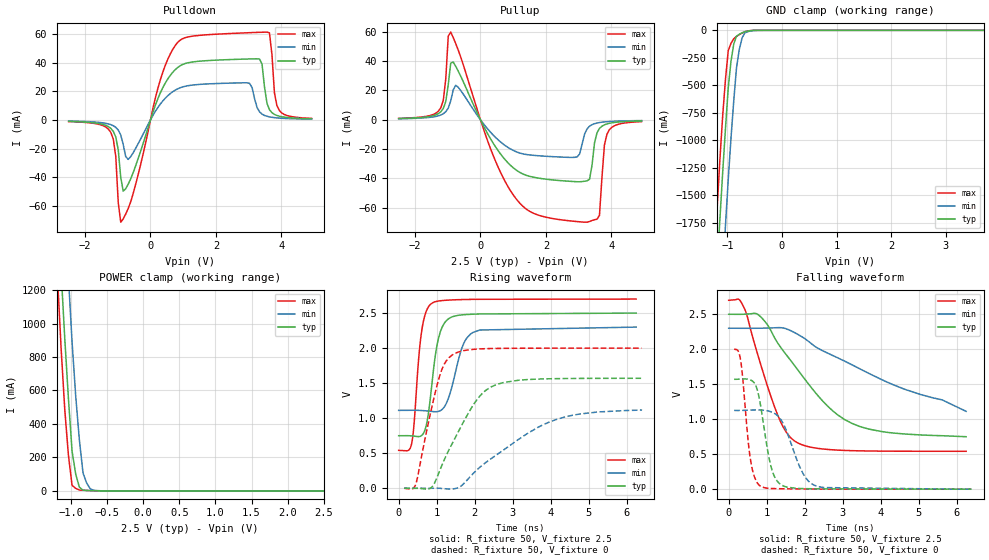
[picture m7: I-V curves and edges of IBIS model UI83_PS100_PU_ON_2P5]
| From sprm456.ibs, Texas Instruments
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|IDG09_OUI83_PS100_PU_OFF_2P75; BUFFER IN NORMAL MODE WITH PULLUP AND PU
|LLDOWN OFF
|   Model Cell UI83_PS100_PU_ON_2P5
|IDG09_OUI83_PS100_PU_ON_2P5
[Model]   UI83_PS100_PU_ON_2P5
Model_type   I/O
Polarity   Non-Inverting
Enable   Active-Low
Vinl =  0.7V
Vinh =  1.7V
Cref =  15pF
Rref =  100.00M
Vref =  0V
Vmeas =  1.25
C_comp   4.785p   4.743p   5.018p
[Model Spec]
Vinl   0.7V   0.7V   0.7V
Vinh   1.7V   1.7V   1.7V
[Temperature Range]   25   125   -40
[Voltage Range]   2.5   2.3   2.7
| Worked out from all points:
|   slope of the pulldown table from 0 to 0.375 V, typ, clamps not added: 16.7 ohm
|   slope of the pullup table from 0 to 0.375 V, typ, clamps not added: 24.3 ohm
|   GND clamp passes 1 mA (typ) near -0.53 V on its own axis
|   POWER clamp passes 1 mA (typ) near -0.67 V on its own axis
|   rising waveform, R_fixture 50, V_fixture 2.5: 20-80 % time 263ps typ, 360ps min, 200ps max; typ from 0.75 V to 2.5 V
|   rising waveform, R_fixture 50, V_fixture 0: 20-80 % time 922ps typ, 1.79ns min, 495ps max; typ from 0 V to 1.57 V
|   falling waveform, R_fixture 50, V_fixture 2.5: 20-80 % time 1.56ns typ, 2.86ns min, 775ps max; typ from 2.5 V to 0.75 V
|   falling waveform, R_fixture 50, V_fixture 0: 20-80 % time 300ps typ, 487ps min, 213ps max; typ from 1.57 V to 0 V
| Nom Voltages:
|   VDD=1.1, VDDS=2.5, VSS=0, VSSS=0
| Min Voltages:
|   VDD=1, VDDS=2.3, VSS=0, VSSS=0
| Max Voltages:
|   VDD=1.2, VDDS=2.7, VSS=0, VSSS=0
[POWER_clamp]
|   voltage   I(typ)   I(min)   I(max)
-2.5V     14.33A     15.07A     13.92A
-1.187V   1.745A     2.55A      1.279A
-1.136V   1.31A      2.108A     850.1mA
-1.086V   910.1mA    1.685A     485.5mA
-1.035V   552.6mA    1.279A     213.3mA
-984.8mV  237.5mA    889.6mA    33.3mA
-934.3mV  99.9mA     565.9mA    15.21mA
-883.8mV  22.21mA    305.1mA    5.394mA
-833.3mV  4.4mA      107.3mA    3.844mA
-732.3mV  1.653mA    12.24mA    2.077mA
-681.8mV  1.081mA    2.967mA    1.344mA
2.5V      -62.22uA   -39.52uA   -107.1uA
[Pulldown]
|   voltage   I(typ)   I(min)   I(max)
-2.5V     -1.029mA   -780.5uA   -1.158mA
-1.212V   -5.915mA   -3.318mA   -8.754mA
-1.061V   -11.95mA   -5.187mA   -25.54mA
-909.1mV  -40.09mA   -10.52mA   -71.53mA
-681.8mV  -44.99mA   -27.63mA   -62.02mA
303mV     19mA       11.15mA    28.2mA
984.8mV   38.8mA     23.1mA     56.82mA
3.03V     42.63mA    25.53mA    61mA
3.333V    42.55mA    5.654mA    61.25mA
3.636V    7.154mA    2.123mA    60.83mA
3.864V    3.092mA    1.414mA    10.01mA
4.924V    800.1uA    540.5uA    1.094mA
[Pullup]
|   voltage   I(typ)   I(min)   I(max)
-2.5V     856.4uA    691.1uA    993.5uA
-1.212V   5.469mA    3.267mA    8.206mA
-909.1mV  38.64mA    12.9mA     59.79mA
-681.8mV  33.25mA    22.23mA    47.64mA
984.8mV   -32.38mA   -20.68mA   -50.65mA
2.955V    -42.21mA   -25.24mA   -69.37mA
3.182V    -41.85mA   -9.733mA   -69.79mA
3.333V    -40.49mA   -4.356mA   -69.34mA
3.636V    -5.897mA   -1.881mA   -65.15mA
3.788V    -3.419mA   -1.448mA   -17.24mA
3.939V    -2.377mA   -1.175mA   -6.756mA
4.924V    -777.2uA   -520.7uA   -1.228mA
[GND_clamp]
|   voltage   I(typ)   I(min)   I(max)
-2.5V     -14.77A    -15.66A    -14.27A
-1.237V   -2.604A    -3.547A    -2.05A
-1.187V   -2.151A    -3.09A     -1.601A
-1.136V   -1.705A    -2.638A    -1.162A
-1.035V   -889mA     -1.772A    -443mA
-984.8mV  -521mA     -1.356A    -183.2mA
-934.3mV  -279.7mA   -978.6mA   -118.7mA
-883.8mV  -123.6mA   -639.8mA   -76.1mA
-833.3mV  -52.76mA   -339.6mA   -55.47mA
-732.3mV  -22.91mA   -70.07mA   -24.96mA
-429.3mV  -158.7uA   -473.7uA   -130.9uA
5V        0A         0A         0A
[Ramp]
| variable   typ   min   max
dV/dt_f   1.058093/1.5633404n 0.71845704/2.8620974n  1.3054833/0.77919182n
dV/dt_r 0.94951792/0.92585824n 0.68174694/1.7998433n  1.2076225/0.49653644n
R_load = 50
[Rising Waveform]
R_fixture = 50
V_fixture = 2.5
V_fixture_min = 2.3
V_fixture_max = 2.7
|   time   V(typ)   V(min)   V(max)
0s        749.7mV    1.112V     541.4mV
343.1ps   747.5mV    1.113V     640.5mV
606ps     753.9mV    1.11V      2.245V
750.2ps   960.4mV    1.103V     2.557V
910.8ps   1.665V     1.094V     2.652V
1.045ns   2.132V     1.097V     2.672V
1.197ns   2.351V     1.158V     2.681V
1.68ns    2.475V     2.025V     2.693V
1.951ns   2.484V     2.223V     2.696V
6.25ns    2.5V       2.3V       2.7V
[Rising Waveform]
R_fixture = 50
V_fixture = 0
V_fixture_min = 0
V_fixture_max = 0
|   time   V(typ)   V(min)   V(max)
143.6ps   0V         0V         0V
444.3ps   0V         0V         49.73mV
835.8ps   0V         0V         1.068V
1.045ns   203.7mV    0V         1.54V
1.205ns   412.5mV    -6.008mV   1.775V
1.453ns   684.1mV    -7.719mV   1.916V
2.086ns   1.283V     276.1mV    1.987V
2.591ns   1.483V     482.4mV    1.995V
4.15ns    1.564V     982mV      1.999V
6.394ns   1.57V      1.125V     2V
[Falling Waveform]
R_fixture = 50
V_fixture = 2.5
V_fixture_min = 2.3
V_fixture_max = 2.7
|   time   V(typ)   V(min)   V(max)
0s        2.5V       2.3V       2.7V
259.9ps   2.499V     2.3V       2.715V
411.1ps   2.501V     2.299V     2.587V
774.2ps   2.495V     2.3V       1.906V
1.226ns   2.147V     2.307V     1.15V
1.473ns   1.952V     2.299V     852.6mV
1.756ns   1.75V      2.231V     680.7mV
2.608ns   1.185V     1.944V     567.7mV
3.257ns   937.2mV    1.774V     550mV
6.25ns    749.7mV    1.112V     541.4mV
[Falling Waveform]
R_fixture = 50
V_fixture = 0
V_fixture_min = 0
V_fixture_max = 0
|   time   V(typ)   V(min)   V(max)
143.6ps   1.57V      1.125V     2V
318.1ps   1.574V     1.125V     1.83V
595.8ps   1.555V     1.131V     351.4mV
720.6ps   1.471V     1.133V     121.5mV
844.8ps   1.179V     1.132V     39.46mV
1.134ns   285.6mV    1.101V     9.611mV
1.461ns   41.36mV    909.2mV    5.33mV
1.909ns   9.314mV    274mV      3.042mV
2.274ns   5.385mV    51.62mV    2.102mV
6.394ns   0V         0V         0V
